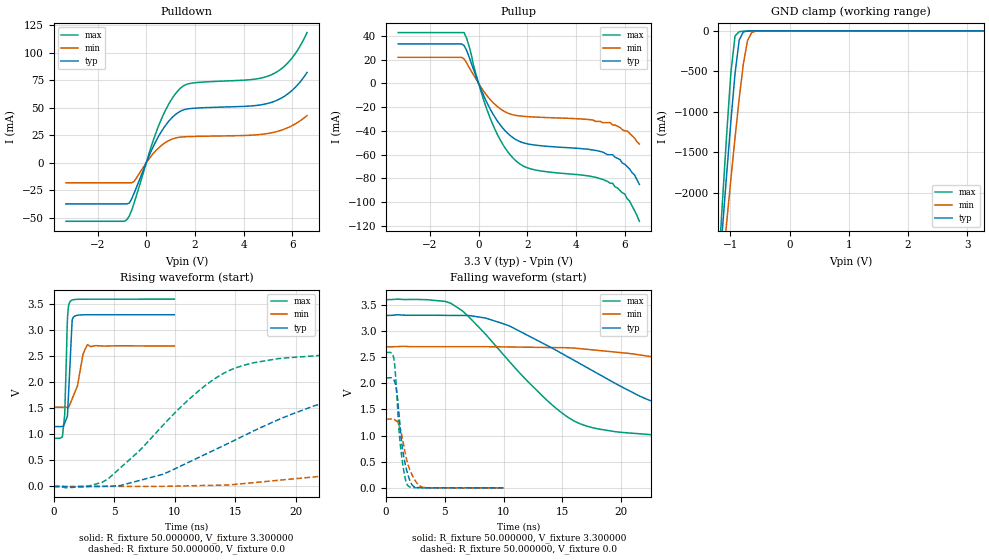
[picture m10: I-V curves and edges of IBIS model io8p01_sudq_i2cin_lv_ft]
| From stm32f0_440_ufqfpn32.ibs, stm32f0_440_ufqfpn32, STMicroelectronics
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|   Model io8p01_sudq_i2cin_lv_ft
[Model]  io8p01_sudq_i2cin_lv_ft
Model_type I/O
Polarity   Non-Inverting
Enable   Active-Low
Vinl =   0.990000V
Vinh =   2.310000V
Vmeas =  1.650000V
Cref =   50.000000pF
Rref =   100.000000M
Vref =   0.0V
C_comp   2.070000pF   1.996000pF   2.160200pF
[Temperature Range]   25.000000   0.125000k   -40.000000
[Pullup Reference]   3.300000V   2.700000V   3.600000V
[Pulldown Reference]   0.0V   0.0V   0.0V
[POWER Clamp Reference]   3.300000V   2.700000V   3.600000V
[GND Clamp Reference]   0.0V   0.0V   0.0V
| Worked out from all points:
|   slope of the pulldown table from 0 to 0.495 V, typ, clamps not added: 20.9 ohm
|   slope of the pullup table from 0 to 0.495 V, typ, clamps not added: 22.2 ohm
|   GND clamp passes 1 mA (typ) near -0.64 V on its own axis
|   rising waveform, R_fixture 50.000000, V_fixture 3.300000: 20-80 % time 272ps typ, 710ps min, 191ps max; typ from 1.15 V to 3.3 V
|   rising waveform, R_fixture 50.000000, V_fixture 0.0: 20-80 % time 12.7ns typ, 30.6ns min, 7.05ns max; typ from 0 V to 2.1 V
|   falling waveform, R_fixture 50.000000, V_fixture 3.300000: 20-80 % time 11ns typ, 22.9ns min, 6.88ns max; typ from 3.3 V to 1.15 V
|   falling waveform, R_fixture 50.000000, V_fixture 0.0: 20-80 % time 671ps typ, 889ps min, 549ps max; typ from 2.1 V to 0 V
[Pulldown]
|Voltage   I(typ)   I(min)   I(max)
-3.3V     -37.45mA   -18.2mA    -53.24mA
-800mV    -37.45mA   -18.2mA    -51.9mA
-700mV    -36.7mA    -18.2mA    -48.48mA
-500mV    -27.71mA   -17.01mA   -36.66mA
200mV     10.57mA    6.084mA    14.57mA
500mV     23.91mA    13.38mA    33.24mA
900mV     37.17mA    19.87mA    52.48mA
1.3V      45.55mA    23.01mA    65.5mA
1.8V      49.29mA    23.83mA    72.18mA
5.1V      54.68mA    27.07mA    79.72mA
5.9V      64.2mA     32.82mA    93.01mA
6.6V      82.13mA    42.97mA    118.4mA
[Pullup]
|Voltage   I(typ)   I(min)   I(max)
-3.3V     33.16mA    21.89mA    42.7mA
-600mV    31.87mA    20.58mA    42.7mA
-400mV    22.79mA    13.76mA    31.9mA
100mV     -5.13mA    -3.299mA   -6.952mA
500mV     -22.5mA    -14.16mA   -30.52mA
900mV     -35.28mA   -21.55mA   -48mA
1.4V      -45.54mA   -26.4mA    -62.53mA
2.2V      -51.57mA   -28.22mA   -72.25mA
4.6V      -55.8mA    -30.6mA    -78.19mA
5.5V      -60mA      -35mA      -84mA
6V        -68mA      -40mA      -93mA
6.6V      -85mA      -51mA      -116mA
[GND_clamp]
|Voltage   I(typ)   I(min)   I(max)
-3.3V     -9.366A    -9.678A    -9.859A
-1.2V     -3.091A    -3.431A    -2.911A
-1.13V    -2.415A    -2.888A    -2.072A
-1.06V    -1.751A    -2.352A    -1.259A
-990mV    -1.112A    -1.826A    -509.3mA
-920mV    -522.9mA   -1.315A    -61.61mA
-850mV    -112.5mA   -833.8mA   -10.22mA
-780mV    -13.59mA   -408.1mA   -5.256mA
-710mV    -3.081mA   -122.1mA   -2.635mA
-640mV    -945.2uA   -21.36mA   -905.7uA
-570mV    -199.6uA   -4.142mA   -156.8uA
3.28V     0A         0A         0A
[POWER_clamp]
|Voltage   I(typ)   I(min)   I(max)
-3.28V    0A         0A         0A
0V        0A         0A         0A
[Ramp]
| variable   typ   min   max
dV/dt_r  1.26216/12.63809n   0.78954/30.54149n   1.55442/7.04027n
dV/dt_f  1.28952/10.87049n   0.70680/22.89628n   1.60469/6.86768n
R_load = 50.000000
[Rising Waveform]
R_fixture= 50.000000
V_fixture= 3.300000
V_fixture_min= 2.700000
V_fixture_max= 3.600000
|time   V(typ)   V(min)   V(max)
0s        1.151V     1.522V     925.5mV
720.7ps   1.153V     1.522V     978.1mV
900.9ps   1.221V     1.521V     1.381V
1.121ns   1.346V     1.522V     3.18V
1.201ns   1.702V     1.522V     3.439V
1.361ns   2.459V     1.594V     3.559V
1.522ns   3.204V     1.686V     3.583V
2.422ns   3.298V     2.547V     3.598V
2.783ns   3.3V       2.725V     3.598V
9.97ns    3.3V       2.7V       3.6V
[Rising Waveform]
R_fixture= 50.000000
V_fixture= 0.0
V_fixture_min= 0.0
V_fixture_max= 0.0
|time   V(typ)   V(min)   V(max)
0s        1.669nV    11.1nV     2.206nV
4.505ns   5.504mV    256.3nV    148.8mV
9.009ns   233.4mV    1.738mV    1.171V
14.51ns   837.7mV    28.62mV    2.229V
23.52ns   1.69V      227.1mV    2.541V
29.53ns   1.939V     389.6mV    2.57V
37.54ns   2.047V     632.6mV    2.587V
57.06ns   2.096V     1.074V     2.592V
82.08ns   2.104V     1.27V      2.591V
249.2ns   2.104V     1.316V     2.591V
[Falling Waveform]
R_fixture= 50.000000
V_fixture= 3.300000
V_fixture_min= 2.700000
V_fixture_max= 3.600000
|time   V(typ)   V(min)   V(max)
0s        3.3V       2.7V       3.6V
5.506ns   3.3V       2.701V     3.533V
10.01ns   3.138V     2.697V     2.542V
13.51ns   2.747V     2.687V     1.713V
16.02ns   2.438V     2.675V     1.277V
23.52ns   1.578V     2.477V     1V
29.03ns   1.337V     2.283V     964.6mV
39.54ns   1.214V     1.9V       935.9mV
59.06ns   1.166V     1.636V     926.5mV
249.2ns   1.151V     1.522V     925.5mV
[Falling Waveform]
R_fixture= 50.000000
V_fixture= 0.0
V_fixture_min= 0.0
V_fixture_max= 0.0
|time   V(typ)   V(min)   V(max)
0s        2.104V     1.316V     2.591V
660.7ps   2.062V     1.315V     2.467V
900.9ps   1.844V     1.273V     1.809V
1.081ns   1.441V     1.206V     1.143V
1.221ns   1.088V     1.114V     792.8mV
1.562ns   519.5mV    733.7mV    248.3mV
1.882ns   228.2mV    429.2mV    34.48mV
2.342ns   25.81mV    187.8mV    4.303mV
3.083ns   2.305mV    13.06mV    1.329mV
9.97ns    1.669nV    11.1nV     2.206nV
